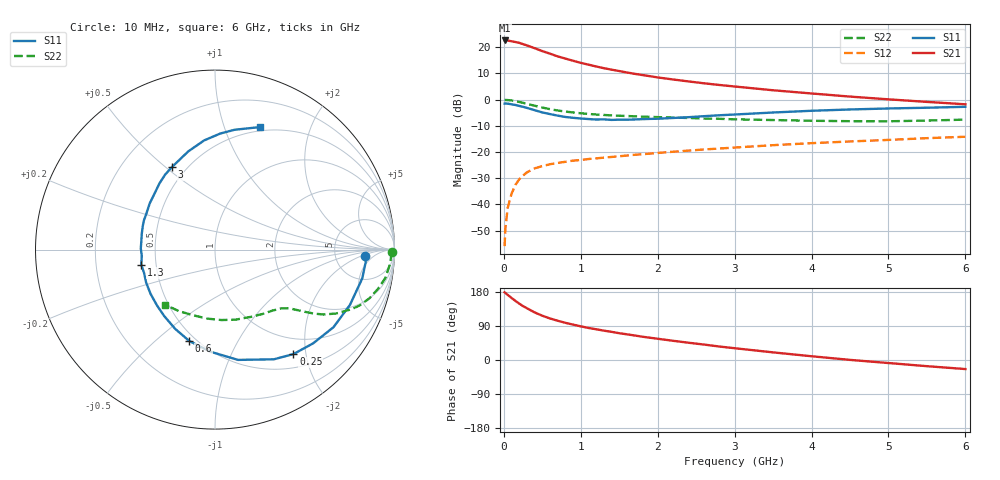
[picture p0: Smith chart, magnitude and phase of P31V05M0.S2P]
! SIEMENS Small Signal Semiconductors
! BFP181
! Si NPN RF Bipolar Junction Transistor in SOT143
! VCE = 1 V  IC = 5 mA
! Common Emitter S-Parameters:  March  1996
# GHz  S  MA  R  50
!  f  S11  S21  S12  S22
! GHz  MAG  ANG  MAG  ANG  MAG  ANG  MAG  ANG
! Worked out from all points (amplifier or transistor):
!   36 points, 10 MHz to 6 GHz, reference 50 ohm
!   highest |S21| = 22.5 dB at 10 MHz (marker M1)
!   |S21| within 3 dB of that: start of sweep to 405.1 MHz
!   unconditionally stable (mu >= 1): 1.361 GHz to end of sweep
!   at 250 MHz: K = 0.25, MSG = 25.1 dB, |S12| = -29.0 dB
!   at 1.4 GHz: K = 1.02, MAG = 15.8 dB, |S12| = -21.9 dB
!   at 6 GHz: K = 1.12, MAG = 4.1 dB, |S12| = -14.2 dB
!   S11 on the Smith chart (normalised r, x): 10 MHz: 11, -3; 250 MHz: 0.72, -1.78; 600 MHz: 0.46, -0.65; 1.3 GHz: 0.41, -0.08; 3 GHz: 0.42, +0.53; 6 GHz: 0.46, +1.33
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0.01  0.8377 -2.4  13.41 178.5  0.0016 83.9  0.984 -0.9
0.02  0.8425 -4.7  13.39 177.2  0.0035 87.5  0.9831 -1.9
0.05  0.8359 -11.1  13.33 171.8  0.0086 87.1  0.978 -4.8
0.1  0.8126 -22.3  12.96 163.8  0.016 77.2  0.9627 -9.4
0.15  0.7891 -33.2  12.53 156.1  0.0235 71.6  0.9338 -13.6
0.2  0.7564 -43.6  12.08 148.8  0.0302 68.0  0.903 -17.4
0.25  0.728 -53.1  11.41 142.1  0.0355 62.6  0.8663 -20.9
0.3  0.6936 -61.8  10.79 136.6  0.0409 58.7  0.83 -23.6
0.4  0.6278 -78.2  9.555 125.6  0.0486 53.1  0.7632 -27.8
0.5  0.5689 -92.8  8.4 116.8  0.0541 48.1  0.7042 -30.9
0.6  0.5286 -105.8  7.509 109.6  0.0584 45.1  0.6561 -32.9
0.7  0.494 -116.8  6.66 103.6  0.062 42.8  0.6191 -34.3
0.8  0.4657 -127.5  6.048 98.1  0.065 41.1  0.5906 -35.4
1.1  0.4253 -154.5  4.636 84.6  0.0735 38.6  0.5316 -38.1
1.3  0.4195 -168.4  3.97 77.5  0.0781 37.4  0.5089 -40.0
1.7  0.4174 167.8  3.096 64.7  0.0885 36.7  0.4794 -44.1
2.2  0.4456 144.7  2.416 50.7  0.1012 35.1  0.4537 -50.7
3  0.5188 117.5  1.776 31.1  0.1216 31.7  0.4201 -63.8
3.5  0.5667 105.3  1.505 20.1  0.135 29.2  0.4069 -73.7
4.5  0.6474 87.4  1.14 0.3  0.1589 22.8  0.387 -96.7
5.5  0.699 75.0  0.903 -16.3  0.1836 16.7  0.3975 -120.5
6  0.7281 69.7  0.813 -23.9  0.1955 13.0  0.4146 -132.3
